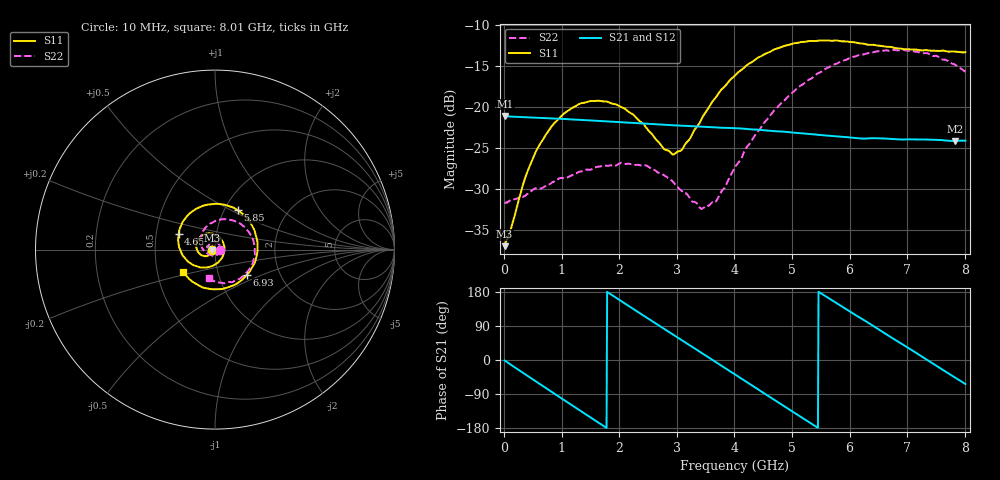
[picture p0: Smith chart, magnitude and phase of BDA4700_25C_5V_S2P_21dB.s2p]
!Agilent Technologies,E5071B,MY42404982,A.09.10
!Date: Mon Oct 20 13:36:55 2025
!Data & Calibration Information:
!Freq	S11:SOLT2(ON)	S21:SOLT2(ON)	S12:SOLT2(ON)	S22:SOLT2(ON)
# Hz S RI R 50
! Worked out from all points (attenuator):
!   801 points, 10 MHz to 8.01 GHz, reference 50 ohm
!   highest |S21| = -21.09 dB at 20 MHz (marker M1); lowest = -24.1 dB at 7.83 GHz (marker M2)
!   lowest |S11| = -37.0 dB at 10 MHz (marker M3), VSWR 1.03, Z = 48.6 - j0.142 ohm
!   |S11| at or under -10 dB: start of sweep to end of sweep
!   |S22| runs from -32.4 to -13.0 dB; largest |S21 - S12| = 0.00067
!   S11 on the Smith chart (normalised r, x): 10 MHz: 0.97, -0.00; 4.65 GHz: 0.65, +0.12; 5.85 GHz: 1.15, +0.54; 6.93 GHz: 1.36, -0.40; 8.01 GHz: 0.68, -0.17
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1e7  -0.0141 -0.00146  0.0882 -0.00193  0.0882 -0.00199  0.0261 -0.000802
2e7  -0.0145 -0.00221  0.0882 -0.00334  0.0881 -0.00366  0.026 -0.00109
3.6e8  -0.0253 -0.0262  0.0694 -0.0523  0.0694 -0.0523  0.022 -0.0184
5.8e8  -0.0427 -0.0361  0.0442 -0.0741  0.0442 -0.074  0.0139 -0.0288
9.9e8  -0.0845 -0.0243  -0.0154 -0.0835  -0.0154 -0.0835  -0.0144 -0.034
1.35e9  -0.1048 0.0157  -0.0606 -0.0575  -0.0607 -0.0576  -0.0366 -0.0176
2.06e9  -0.0417 0.0903  -0.072 0.0369  -0.072 0.0369  -0.0306 0.0338
2.68e9  0.0441 0.0427  -0.00262 0.0784  -0.00263 0.0784  0.0142 0.0371
2.92e9  0.0518 1.96e-05  0.0285 0.0721  0.0285 0.0721  0.0256 0.0244
3.06e9  0.047 -0.0268  0.0446 0.063  0.0442 0.0632  0.0283 0.0135
3.44e9  -0.00445 -0.0861  0.0725 0.0232  0.0726 0.0231  0.0184 -0.0154
3.69e9  -0.0597 -0.1  0.0747 -0.00879  0.0748 -0.00897  -0.000323 -0.0269
4.01e9  -0.1361 -0.0764  0.0586 -0.046  0.0586 -0.0459  -0.0334 -0.0265
4.65e9  -0.2025 0.0888  -0.0138 -0.0702  -0.0136 -0.0703  -0.0805 0.0442
5.35e9  -0.049 0.2488  -0.0672 -0.0127  -0.0672 -0.0129  -0.0156 0.1499
5.85e9  0.1262 0.2191  -0.0525 0.04  -0.0524 0.0401  0.0982 0.163
6.25e9  0.2207 0.1045  -0.0169 0.062  -0.0162 0.0622  0.1823 0.1053
6.68e9  0.2264 -0.0583  0.0283 0.0575  0.0284 0.0575  0.2212 -0.00242
6.93e9  0.178 -0.1399  0.0484 0.041  0.0486 0.0408  0.2123 -0.072
7.37e9  0.0308 -0.2202  0.0634 -0.00219  0.0633 -0.00231  0.1347 -0.1642
7.83e9  -0.1342 -0.1731  0.0432 -0.0447  0.0432 -0.0449  0.00985 -0.1817
8.01e9  -0.1789 -0.1225  0.0278 -0.0559  0.028 -0.0559  -0.0339 -0.1609
